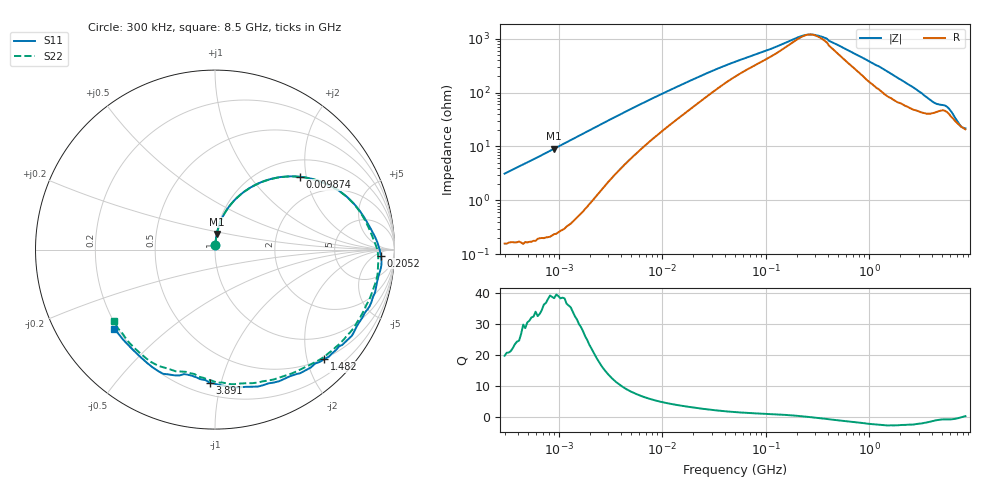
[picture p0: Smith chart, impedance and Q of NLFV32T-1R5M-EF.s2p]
! S-parameter Generated by TDK Corporation
! Copyright(C) 2015 TDK Corporation.
! All Rights Reserved.
! TDK P/N: NLFV32T-1R5M-EF (Inductors)
! Property: L=1.5uH at 7.96MHz
! Size(LxWxT): 3.2x2.5x2.2mm, 0.126x0.098x0.087inches
! Model Type: s2p (Touchstone File Format Version 1.0)
! Frequency: DC=Yes Start=0.3MHz Stop=8500MHz 225points Log-sweep
! Note:
! Model Generated on Jun. 23, 2015
! Hash(MD5):
! Port Assignments:
!  1 ---@@@--- 2
! Applicable Conditions:
!  Temperature = 25 degC
!  DC Bias Current = 0 A
!  Small Signal Operation
! Terms and conditions regarding TDK Simulation Models
! (1)This simulation model is being provided solely for informational purposes. Please refer to the specifications of the products in terms of detailed characteristics of such products.
! (2)In no event shall TDK Corporation of any of its subsidiaries be liable for any loss or damage arising, directly or indirectly,
!  From any information contained in this simulation model, including, but not limited to loss or damages arising from any inaccuracies, omissions or errors in connection with such information.
! (3)Any and all copyrights on this simulation model are owned by TDK Corporation.
!  Duplication or redistribution of this simulation model without prior written permission from TDK Corporation is prohibited.
! (4)This simulation model is subject to any modification or change without any prior notice.
! (5)Neither TDK Corporation nor any of its subsidiaries shall make any warranty, express or implied,
!  Including but not limited to the correctness, implied warranties of merchantability and fitness for a particular purpose with respect to this simulation models.
! (6)The use of this simulation model shall be deemed to have consented to the terms and conditions hereof.
# MHz S MA R 50
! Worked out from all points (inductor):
!   224 points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, 300 kHz to 8.5 GHz, reference 50 ohm
!   read as one part in series: L = 1.64 uH near 314.1 kHz
!   highest Q = 39 at 904.3 kHz (marker M1), where L = 1.6 uH
!   self-resonance near 266.1 MHz
!   S11 on the Smith chart (normalised r, x): 300 kHz: 1.00, +0.06; 9.874 MHz: 1.38, +1.84; 205.2 MHz: 21, -10; 1.482 GHz: 0.49, -2.33; 3.891 GHz: 0.28, -0.92; 8.5 GHz: 0.19, -0.33
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0.3  0.02826 85.9  0.9962 -1.7  0.9993 -2.2  0.02825 85.9
0.9042579  0.08812 83.5  0.9929 -5.1  0.995 -5.5  0.08813 83.4
1.72111  0.1676 78.3  0.9791 -9.6  0.9815 -10.1  0.1677 78.2
3.937196  0.354 63.9  0.9018 -20.6  0.9036 -21.1  0.3541 63.7
9.430415  0.6117 41.7  0.6811 -37.0  0.6823 -37.4  0.6121 41.6
9.874071  0.6241 40.6  0.6663 -37.8  0.6675 -38.2  0.6244 40.5
22.58783  0.7904 22.0  0.4047 -48.6  0.4053 -49.0  0.7902 21.8
51.67171  0.8612 10.1  0.2285 -47.5  0.2289 -47.9  0.8567 9.9
205.2186  0.9249 -2.1  0.08705 -22.8  0.08722 -23.3  0.9105 -2.6
283.1228  0.9306 -5.8  0.07762 -0.3  0.07777 -0.7  0.9137 -6.3
390.6008  0.9219 -10.3  0.09176 21.4  0.09204 20.9  0.9141 -10.7
778.4218  0.9044 -24.8  0.1765 35.9  0.1766 35.5  0.8926 -25.1
1025.67  0.9013 -32.1  0.2237 34.3  0.2233 33.8  0.8772 -33.1
1481.602  0.8621 -45.0  0.295 25.9  0.2957 24.9  0.8462 -46.5
1551.304  0.8561 -46.9  0.3051 24.4  0.3058 23.3  0.8397 -48.2
2693.286  0.7999 -72.5  0.4049 -0.2  0.4047 -1.6  0.7727 -74.4
3890.506  0.7416 -92.3  0.4475 -22.6  0.4486 -23.4  0.7254 -93.1
5126.239  0.715 -104.0  0.4151 -42.0  0.4151 -42.5  0.7042 -105.2
5884.306  0.7417 -110.3  0.397 -47.6  0.3994 -47.9  0.7205 -115.8
6450.987  0.7471 -115.1  0.4043 -51.8  0.4071 -52.2  0.7137 -124.8
7404.957  0.7291 -124.4  0.4179 -61.7  0.4193 -62.7  0.696 -137.7
8500  0.7131 -141.9  0.3975 -78.6  0.3968 -78.0  0.6896 -144.8
